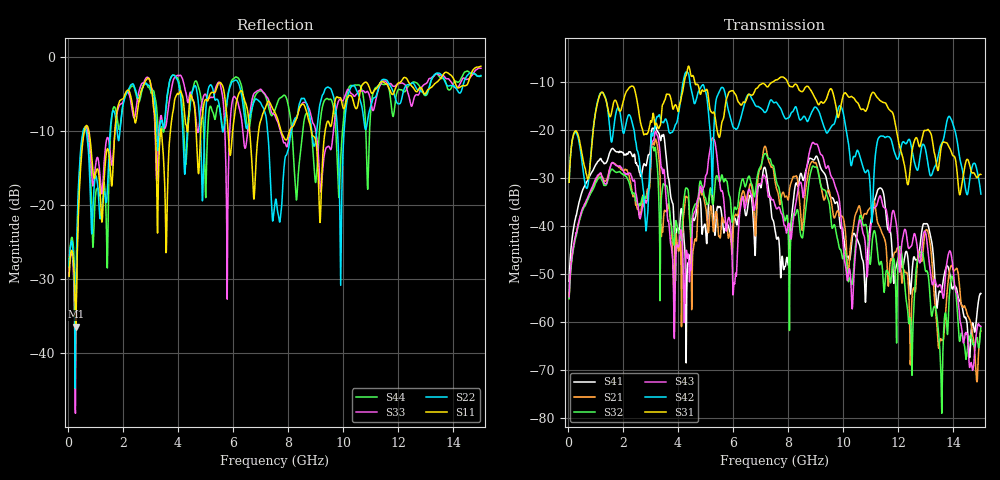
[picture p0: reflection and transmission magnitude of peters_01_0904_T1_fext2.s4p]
# MHZ S RI R 50.00
! FREQ  S11  S12  S13  S14
!  S21  S22  S23  S24
!  S31  S32  S33  S34
!  S41  S42  S43  S44
!  REAL  IMAG  REAL  IMAG  REAL  IMAG  REAL  IMAG
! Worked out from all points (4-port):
!   1496 points, 50 MHz to 15 GHz, reference 50 ohm
!   strongest paths, dB at 50 MHz, 3.79 GHz, 7.53 GHz, 11.27 GHz, 15 GHz:
!     S31: -30.9, -14.8, -9.7, -13.5, -29.3
!     S42: -30.9, -20.5, -14.3, -21.9, -33.4
!     S43: -54.8, -45.8, -35.8, -34.7, -61.0
!     S32: -55.2, -41.3, -29.3, -46.8, -61.1
!     S21: -55.1, -43.2, -30.9, -39.6, -62.0
!     S41: -51.6, -35.1, -41.0, -32.4, -54.1
!   lowest |S11| = -36.4 dB at 290 MHz (marker M1), VSWR 1.03, Z = 51.5 + j0.275 ohm
!   |S11| at or under -10 dB: start of sweep to 605.1 MHz; 767.5 MHz to 1.714 GHz (946.2 MHz wide, 76.3 % of centre); 8.842 GHz to 9.345 GHz (503 MHz wide, 5.53 % of centre)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
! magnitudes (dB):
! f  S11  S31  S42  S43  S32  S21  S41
! 50 MHz  -29.6  -30.9  -30.9  -54.8  -55.2  -55.1  -51.6
! 290 MHz  -36.4  -20.2  -20.5  -41.9  -42.4  -42.1  -38.2
! 2.86 GHz  -3.1  -21.0  -40.3  -35.2  -34.1  -33.6  -27.2
! 4.34 GHz  -10.1  -7.5  -8.0  -46.4  -32.3  -34.1  -49.2
! 8.95 GHz  -10.8  -13.1  -15.4  -22.9  -27.8  -26.9  -26.2
! 10.32 GHz  -5.4  -13.1  -27.0  -57.1  -52.3  -42.0  -42.9
! 15 GHz  -1.3  -29.3  -33.4  -61.0  -61.1  -62.0  -54.1
